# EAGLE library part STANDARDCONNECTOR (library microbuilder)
Standard 20-Pin MCU Connector
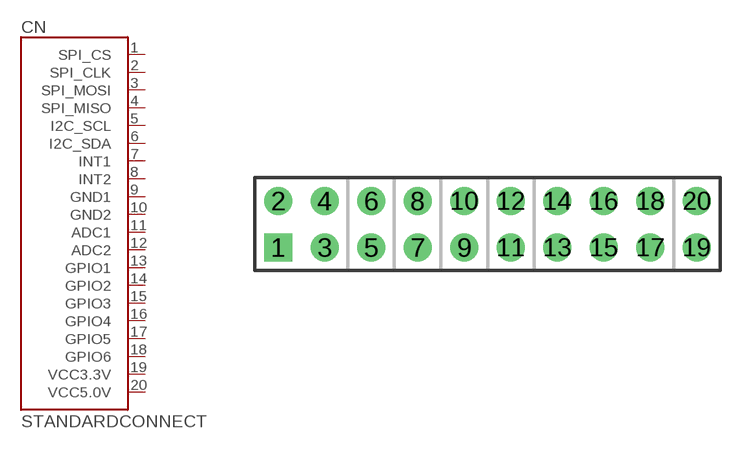
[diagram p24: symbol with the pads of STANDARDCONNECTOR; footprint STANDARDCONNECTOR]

Designator prefix CN

## STANDARDCONNECTOR  [STANDARDCONNECTOR]
1  SPI_CS
2  SPI_CLK
3  SPI_MOSI
4  SPI_MISO
5  I2C_SCL
6  I2C_SDA
7  INT1
8  INT2
9  GND1
10  GND2
11  ADC1
12  ADC2
13  GPIO1
14  GPIO2
15  GPIO3
16  GPIO4
17  GPIO5
18  GPIO6
19  VCC3.3V
20  VCC5.0V

## Footprint STANDARDCONNECTOR (pad centres in mm)
drill 1 square: 1 -11.43,-1.27
drill 1: 2 -11.43,1.27; 3 -8.89,-1.27; 4 -8.89,1.27; 5 -6.35,-1.27; 6 -6.35,1.27; 7 -3.81,-1.27; 8 -3.81,1.27; 9 -1.27,-1.27; 10 -1.27,1.27; 11 1.27,-1.27; 12 1.27,1.27; 13 3.81,-1.27; 14 3.81,1.27; 15 6.35,-1.27; 16 6.35,1.27; 17 8.89,-1.27; 18 8.89,1.27; 19 11.43,-1.27; 20 11.43,1.27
